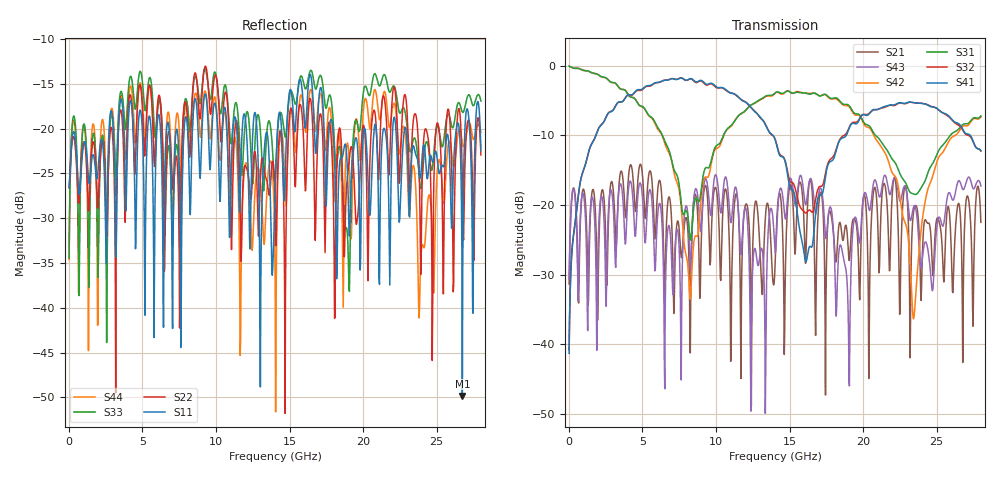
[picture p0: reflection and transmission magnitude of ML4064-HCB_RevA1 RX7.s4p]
! TOUCHSTONE file generated by CST DESIGN STUDIO
! Date and time: Wed Aug 26 10:45:14 2020
! Project name:  Project name: C:\Users\Simulation2\Temp\DE66\Untitled_0.cst
! Tree item: Tasks\SPara1\S-Parameters
# GHz S MA R 50
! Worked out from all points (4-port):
!   1000 points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, 28 MHz to 28 GHz, reference 50 ohm
!   strongest paths, dB at 28 MHz, 7.028 GHz, 14.03 GHz, 21.03 GHz, 28 GHz:
!     S41: -41.3, -1.9, -10.6, -6.3, -12.2
!     S32: -40.8, -1.9, -10.6, -6.2, -12.3
!     S31: -0.1, -13.9, -3.9, -10.4, -7.2
!     S42: -0.1, -14.0, -4.0, -11.0, -7.3
!     S43: -30.7, -30.4, -26.9, -18.2, -17.3
!     S21: -31.4, -24.4, -28.1, -25.2, -22.5
!   lowest |S11| = -49.8 dB at 26.74 GHz (marker M1), VSWR 1.01, Z = 49.7 - j0.167 ohm
!   |S11| at or under -10 dB: start of sweep to end of sweep
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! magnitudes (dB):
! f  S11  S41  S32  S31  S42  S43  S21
! 28 MHz  -26.6  -41.3  -40.8  -0.1  -0.1  -30.7  -31.4
! 4.62 GHz  -25.5  -3.5  -3.6  -5.2  -5.1  -21.4  -19.0
! 8.232 GHz  -28.9  -1.9  -1.9  -24.6  -33.2  -27.3  -37.9
! 16.13 GHz  -19.1  -28.1  -21.2  -4.0  -3.9  -19.8  -26.6
! 23.44 GHz  -22.0  -5.3  -5.3  -18.4  -36.3  -20.2  -20.9
! 26.74 GHz  -49.8  -9.0  -9.2  -8.5  -8.8  -17.7  -34.6
! 28 GHz  -22.5  -12.2  -12.3  -7.2  -7.3  -17.3  -22.5
